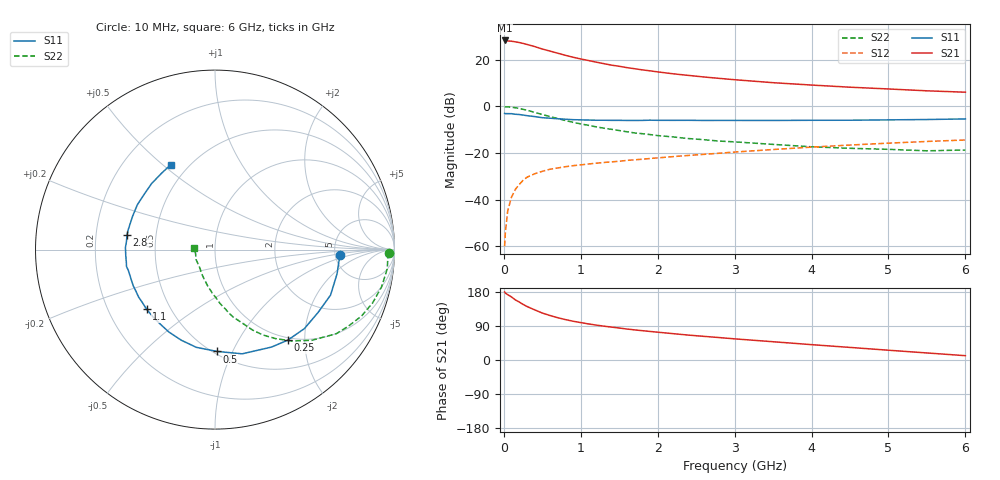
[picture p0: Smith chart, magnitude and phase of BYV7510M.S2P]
! SIEMENS Small Signal Semiconductors
! BFY420
! Si NPN RF SIEGET Grounded Emitter Transistor in MICRO-X
! VCE = 0.75 V  IC = 10 mA
! Common Emitter S-Parameters:  October  1996
# GHz  S  MA  R  50
!  f  S11  S21  S12  S22
! GHz  MAG  ANG  MAG  ANG  MAG  ANG  MAG  ANG
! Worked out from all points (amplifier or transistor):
!   36 points, 10 MHz to 6 GHz, reference 50 ohm
!   highest |S21| = 28.2 dB at 10 MHz (marker M1)
!   |S21| within 3 dB of that: start of sweep to 436.5 MHz
!   unconditionally stable (mu >= 1): 2.352 GHz to end of sweep
!   at 250 MHz: K = 0.20, MSG = 29.3 dB, |S12| = -31.8 dB
!   at 1.4 GHz: K = 0.78, MSG = 20.7 dB, |S12| = -23.9 dB
!   at 6 GHz: K = 1.13, MAG = 8.1 dB, |S12| = -14.5 dB
!   S11 on the Smith chart (normalised r, x): 10 MHz: 5.57, -0.64; 250 MHz: 0.96, -1.66; 500 MHz: 0.52, -0.87; 1.1 GHz: 0.37, -0.33; 2.8 GHz: 0.34, +0.07; 6 GHz: 0.40, +0.53
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0.01  0.6992 -2.4  25.7 179.5  0.001 100.5  0.9688 -1.1
0.02  0.6942 -4.7  25.57 176.6  0.002 88.4  0.9636 -2.3
0.1  0.6919 -21.5  24.76 166.3  0.0113 80.4  0.9512 -12.6
0.15  0.6727 -31.4  23.97 158.6  0.0165 74.6  0.9266 -18.8
0.2  0.6647 -41.5  23.21 153.0  0.021 70.5  0.8963 -24.4
0.25  0.6472 -51.2  22.19 146.7  0.0258 66.2  0.8567 -29.9
0.3  0.6277 -59.9  21.13 141.3  0.03 63.3  0.8226 -34.7
0.4  0.6001 -75.4  19.02 132.4  0.0356 57.4  0.7386 -43.2
0.5  0.5673 -88.9  16.83 123.9  0.0402 53.2  0.6645 -50.0
0.6  0.5544 -100.8  15.2 117.4  0.0446 50.4  0.5996 -55.8
0.7  0.5388 -110.3  13.7 111.6  0.0475 48.5  0.5444 -60.8
0.8  0.5261 -119.3  12.34 106.7  0.0505 46.1  0.4943 -65.0
0.9  0.515 -126.3  11.22 102.3  0.0532 45.2  0.4512 -68.3
1.1  0.5056 -138.9  9.549 95.2  0.0577 44.2  0.389 -74.9
1.3  0.5011 -148.2  8.181 89.3  0.0622 43.0  0.3382 -79.8
1.6  0.4959 -160.1  6.719 81.7  0.069 42.7  0.2836 -87.0
2.2  0.4982 -176.7  4.956 69.5  0.0831 42.0  0.2196 -98.2
2.8  0.4965 170.8  3.956 59.2  0.0983 40.3  0.1789 -108.6
3.5  0.4953 157.8  3.196 48.2  0.118 37.1  0.152 -119.6
4.5  0.5009 141.7  2.558 33.2  0.1471 30.2  0.1253 -136.9
5.5  0.5189 125.2  2.139 18.6  0.1757 21.5  0.1107 -167.6
6  0.5339 117.5  1.998 11.4  0.189 16.9  0.1153 175.7
